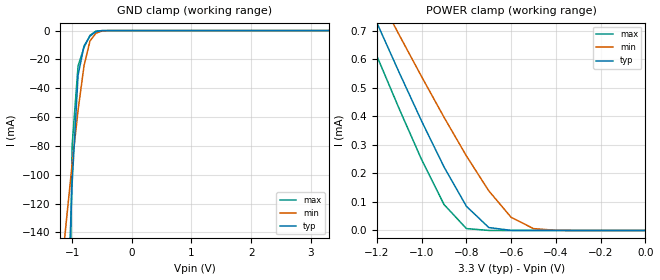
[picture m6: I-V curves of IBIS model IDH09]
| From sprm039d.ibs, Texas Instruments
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[Model]   IDH09
Model_type   Input
Polarity   Non-Inverting
| signals   A, Y
Vinl = 0.8V
Vinh = 2.0V
|   typ   min   max
C_comp   1.5797p   1.5046p   1.7659p
|   typ   min   max
[Temperature Range]   25   -40   125
|   typ   min   max
[Voltage Range]   3.30V   3.00V   3.60V
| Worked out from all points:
|   GND clamp passes 1 mA (typ) near -0.61 V on its own axis
|   POWER clamp passes 1 mA (typ) near -1.35 V on its own axis
[GND_clamp]
|   Voltage   I(typ)   I(min)   I(max)
-3.3V     -3.292A    -1.132A    -11.79A
-1.2V     -345.9mA   -175.9mA   -836.7mA
-1.1V     -219.8mA   -133.6mA   -390.1mA
-1V       -106.6mA   -92.92mA   -80.27mA
-900mV    -31.05mA   -55.3mA    -24.61mA
-800mV    -10.64mA   -24.38mA   -11.61mA
-700mV    -3.852mA   -7.139mA   -3.303mA
-600mV    -739.9uA   -1.804mA   -366.4uA
-500mV    -67.29uA   -326.4uA   -17.03uA
-400mV    -3.755uA   -40.31uA   -379.8nA
3.3V      133.2pA    31.75nA    44.41pA
[POWER_clamp]
|   Voltage   I(typ)   I(min)   I(max)
-3.3V     4.599mA    4.101mA    4.747mA
-1.3V     905.1uA    983.4uA    800.7uA
-1.2V     727.5uA    833.1uA    611.3uA
-1.1V     552.9uA    684.6uA    425.8uA
-1V       383.1uA    538.7uA    248.1uA
-900mV    222.6uA    396.6uA    91.01uA
-800mV    84.79uA    261.3uA    6.786uA
-700mV    10.3uA     138.9uA    73.72nA
-600mV    329.7nA    46.05uA    799.4pA
-500mV    8.393nA    6.46uA     88.82pA
-400mV    399.7pA    466.7nA    44.41pA
0V        1pA        1pA        1pA
